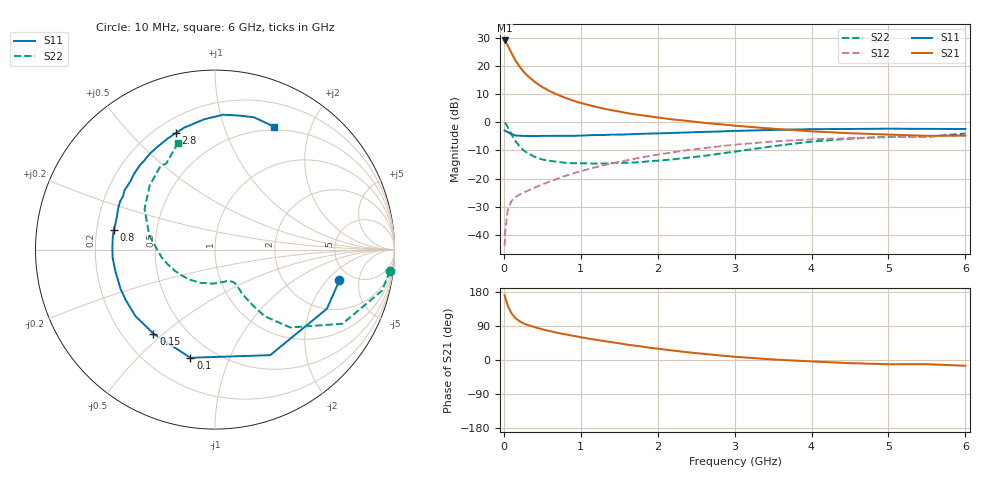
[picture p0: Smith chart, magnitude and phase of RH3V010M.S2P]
! SIEMENS Small Signal Semiconductors
! BFR106
! Si NPN RF Bipolar Junction Transistor in SOT23
! VCE = 3 V  IC = 10 mA
! Common Emitter S-Parameters:  August  1996
# GHz  S  MA  R  50
!  f  S11  S21  S12  S22
! GHz  MAG  ANG  MAG  ANG  MAG  ANG  MAG  ANG
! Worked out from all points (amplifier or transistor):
!   36 points, 10 MHz to 6 GHz, reference 50 ohm
!   highest |S21| = 29.0 dB at 10 MHz (marker M1)
!   |S21| within 3 dB of that: start of sweep to 73.38 MHz
!   unconditionally stable (mu >= 1): 482.7 MHz to 2.143 GHz; 5.052 GHz to end of sweep
!   at 250 MHz: K = 0.71, MSG = 21.6 dB, |S12| = -25.1 dB
!   at 1.4 GHz: K = 1.10, MAG = 7.6 dB, |S12| = -14.7 dB
!   at 6 GHz: K = 1.02, MAG = -0.8 dB, |S12| = -4.7 dB
!   S11 on the Smith chart (normalised r, x): 10 MHz: 3.97, -2.78; 100 MHz: 0.37, -0.73; 150 MHz: 0.33, -0.46; 800 MHz: 0.27, +0.09; 2.8 GHz: 0.28, +0.68; 6 GHz: 0.46, +1.49
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0.01  0.714 -13.9  28.29 171.1  0.0063 85.3  0.9822 -7.0
0.02  0.7054 -27.8  27.51 163.8  0.0123 76.8  0.9585 -13.8
0.05  0.6636 -62.4  23.27 143.6  0.0272 62.6  0.8213 -30.2
0.1  0.618 -102.8  16.89 123.0  0.0401 50.3  0.6031 -46.0
0.15  0.5804 -126.2  12.51 110.5  0.0468 45.9  0.4635 -53.3
0.2  0.5778 -140.2  9.923 103.0  0.0515 45.5  0.3802 -55.7
0.25  0.5711 -150.3  8.087 97.2  0.0558 46.4  0.3211 -57.4
0.3  0.57 -157.4  6.828 93.2  0.0597 47.8  0.2878 -58.3
0.4  0.568 -167.9  5.222 86.7  0.0689 51.2  0.2428 -58.6
0.5  0.5722 -175.4  4.209 81.1  0.0782 54.2  0.218 -59.2
0.6  0.5719 178.6  3.547 76.1  0.089 56.6  0.206 -60.9
0.8  0.5744 169.2  2.701 67.7  0.1115 59.0  0.1903 -66.1
0.9  0.5737 164.4  2.421 63.9  0.1233 59.9  0.1871 -68.5
1.1  0.5864 156.9  2.023 56.6  0.147 60.6  0.1859 -76.7
1.3  0.5927 149.9  1.744 50.0  0.1723 60.2  0.1847 -84.9
1.6  0.607 140.5  1.451 40.7  0.2112 58.4  0.1913 -99.4
2.2  0.6467 123.9  1.119 24.9  0.2935 52.2  0.2192 -130.5
2.8  0.6845 108.7  0.924 12.2  0.3728 43.4  0.276 -162.7
3.5  0.7291 94.6  0.767 1.4  0.4553 31.8  0.3747 167.9
4.5  0.7592 79.5  0.638 -8.3  0.5229 14.9  0.5102 135.5
5.5  0.7611 68.1  0.574 -11.1  0.5531 4.1  0.5514 119.4
6  0.7586 64.2  0.58 -15.2  0.5807 -3.4  0.6302 109.1
